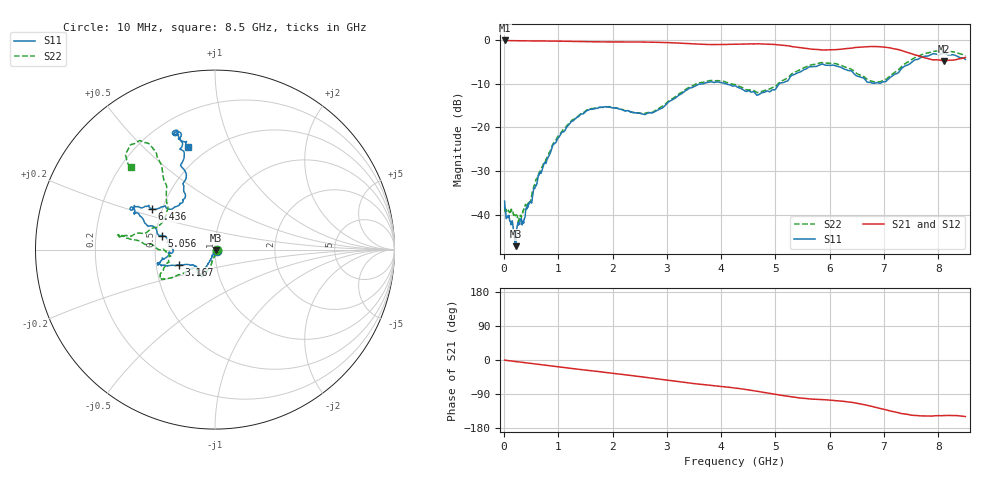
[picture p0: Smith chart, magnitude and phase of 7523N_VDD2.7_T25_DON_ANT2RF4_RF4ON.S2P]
!Agilent Technologies,E5071C,MY46417908,A.11.23
!Date: Wed Dec 09 17:50:21 2020
!Data & Calibration Information:
!Freq	S11:SOLT2(ON)	S21:SOLT2(ON)	S12:SOLT2(ON)	S22:SOLT2(ON)
!PortZ  Port1:50+j0  Port2:50+j0
!Above PortZ is port z conversion or system Z0 setting when saving the data.
!When reading, reference impedance value at option line is always used.
# Hz S dB R 50
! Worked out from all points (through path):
!   1601 points, 10 MHz to 8.5 GHz, reference 50 ohm
!   highest |S21| = -0.17 dB at 10 MHz (marker M1); lowest = -4.8 dB at 8.107 GHz (marker M2)
!   group delay of S21, straight-line fit = 51.3 ps
!   lowest |S11| = -47.1 dB at 211.6 MHz (marker M3), VSWR 1.01, Z = 50.3 - j0.31 ohm
!   |S11| at or under -10 dB: start of sweep to 3.682 GHz; 4.07 GHz to 5.079 GHz (1.009 GHz wide, 22 % of centre)
!   |S22| runs from -41.5 to -2.5 dB; largest |S21 - S12| = 0.0038
!   S11 on the Smith chart (normalised r, x): 10 MHz: 1.03, -0.01; 3.167 GHz: 0.66, -0.12; 5.056 GHz: 0.54, +0.09; 6.436 GHz: 0.44, +0.24; 8.5 GHz: 0.39, +0.69
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1e7  -36.84 -21.0  -0.17 -0.3  -0.17 -0.3  -38.06 -1.3
2.116375e8  -47.11 -44.4  -0.24 -4.0  -0.24 -4.0  -40.19 -41.3
2.912312e8  -41.69 -73.6  -0.24 -5.4  -0.25 -5.4  -40.45 -60.7
4.663375e8  -37.24 -102.0  -0.27 -8.5  -0.27 -8.5  -37.33 -78.5
9.067562e8  -23.91 -112.4  -0.32 -16.3  -0.33 -16.3  -23.69 -102.9
1.426769e9  -16.91 -117.2  -0.42 -25.4  -0.42 -25.4  -16.81 -113.4
1.8778e9  -15.34 -122.8  -0.51 -32.9  -0.51 -32.9  -15.26 -121.8
2.562306e9  -17.01 -136.4  -0.53 -44.9  -0.53 -44.9  -16.85 -134.6
2.843538e9  -15.99 -147.3  -0.59 -50.4  -0.59 -50.4  -15.79 -139.9
3.167219e9  -13.19 -157.2  -0.73 -56.5  -0.73 -56.5  -12.88 -143.6
3.740294e9  -9.77 -165.2  -1.08 -65.8  -1.08 -65.8  -9.44 -150.9
4.255e9  -10.52 -170.7  -1.04 -74.0  -1.03 -74.0  -10.23 -158.9
4.6795e9  -12.59 179.7  -0.94 -82.7  -0.92 -82.8  -12.06 -171.9
5.056244e9  -10.27 165.2  -1.20 -92.1  -1.20 -92.2  -9.95 179.6
5.671769e9  -6.17 155.9  -2.17 -103.2  -2.16 -103.0  -5.72 171.6
6.075044e9  -5.84 151.8  -2.29 -106.9  -2.31 -106.9  -5.39 172.0
6.435869e9  -7.60 147.2  -1.86 -112.4  -1.88 -112.3  -7.08 168.0
6.807306e9  -9.93 129.5  -1.55 -123.4  -1.55 -123.5  -9.59 153.8
7.088538e9  -8.87 118.3  -1.81 -133.4  -1.84 -133.6  -8.51 135.7
7.698756e9  -3.95 107.3  -3.95 -147.6  -3.95 -147.6  -3.38 121.6
8.107338e9  -3.10 109.0  -4.84 -146.6  -4.87 -146.6  -2.51 128.8
8.5e9  -4.53 104.8  -4.05 -149.1  -4.04 -148.9  -3.68 135.4
